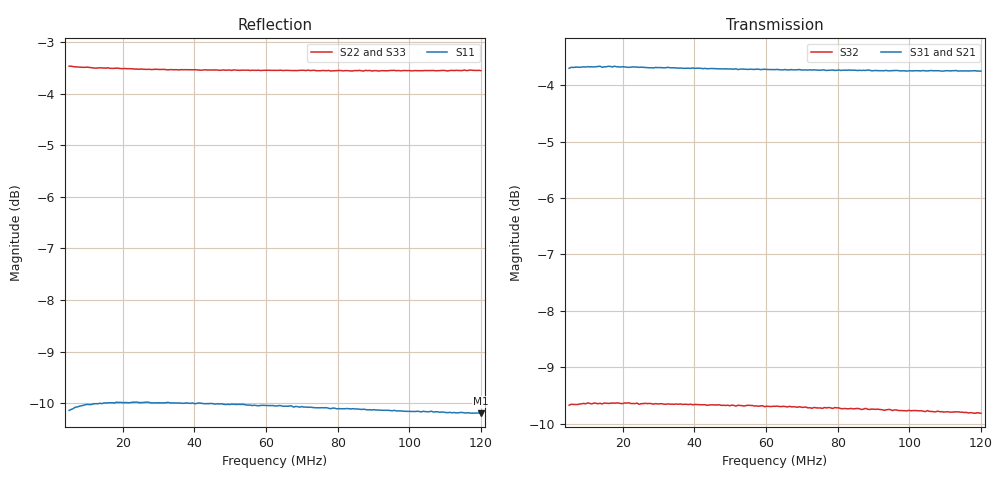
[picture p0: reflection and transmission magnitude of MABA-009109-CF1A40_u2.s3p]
#	MHz	S	RI	R	75
!FREQ	R1	I1	R2	I2	R3	I3
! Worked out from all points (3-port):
!   201 points, 5 MHz to 120 MHz, reference 75 ohm
!   strongest paths, dB at 5 MHz, 33.75 MHz, 62.5 MHz, 91.25 MHz, 120 MHz:
!     S31: -3.7, -3.7, -3.7, -3.7, -3.8
!     S21: -3.7, -3.7, -3.8, -3.8, -3.9
!     S32: -9.7, -9.7, -9.7, -9.7, -9.8
!   lowest |S11| = -10.2 dB at 120 MHz (marker M1), VSWR 1.90, Z = 136 - j24 ohm
!   |S11| at or under -10 dB: start of sweep to 14.46 MHz; 39.71 MHz to 40.83 MHz (1.117 MHz wide, 2.77 % of centre); 41.83 MHz to end of sweep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
5  0.3109 0.0147  0.6539 0.00128  -0.6531 -0.00125
   0.6535 0.00104  -0.6708 0.0105  -0.3287 -0.00304
   -0.6531 -0.00125  -0.3283 -0.00275  -0.6711 0.011
6.725  0.3133 0.00992  0.6546 -0.00385  -0.6545 0.00388
       0.6544 -0.00327  -0.6696 0.0118  -0.3291 -0.0011
       -0.6545 0.00388  -0.3288 -0.00148  -0.67 0.0126
11.325  0.3154 0.00148  0.6549 -0.0125  -0.6549 0.0129
        0.6549 -0.0127  -0.6684 0.015  -0.3292 0.00189
        -0.6549 0.0129  -0.3292 0.00188  -0.668 0.0164
15.925  0.3165 -0.0045  0.6554 -0.0207  -0.6553 0.021
        0.6545 -0.0206  -0.6682 0.0203  -0.3294 0.00449
        -0.6553 0.021  -0.3295 0.00433  -0.6676 0.0207
22.25  0.3166 -0.0112  0.6541 -0.0305  -0.6539 0.0312
       0.6534 -0.0299  -0.6665 0.0245  -0.3299 0.00723
       -0.6539 0.0312  -0.3294 0.00693  -0.6658 0.0259
29.15  0.3161 -0.017  0.6525 -0.0402  -0.6529 0.0414
       0.6519 -0.0409  -0.6656 0.0312  -0.3293 0.00998
       -0.6529 0.0414  -0.3293 0.0103  -0.6648 0.0325
62.5  0.3115 -0.042  0.6425 -0.0855  -0.6452 0.088
      0.6432 -0.0857  -0.6617 0.0623  -0.3268 0.0228
      -0.6452 0.088  -0.3268 0.0224  -0.6575 0.0646
92.975  0.3051 -0.0618  0.6323 -0.1239  -0.6369 0.1285
        0.6314 -0.1247  -0.6579 0.0909  -0.3241 0.0328
        -0.6369 0.1285  -0.3233 0.0327  -0.6511 0.0936
94.7  0.3047 -0.0629  0.6307 -0.1255  -0.6365 0.1307
      0.6308 -0.1269  -0.658 0.0925  -0.323 0.0336
      -0.6365 0.1307  -0.3237 0.0334  -0.6507 0.0952
120  0.2988 -0.0796  0.6195 -0.1566  -0.6284 0.1632
     0.6185 -0.1577  -0.6542 0.1149  -0.3203 0.041
     -0.6284 0.1632  -0.3204 0.0408  -0.6429 0.1174
